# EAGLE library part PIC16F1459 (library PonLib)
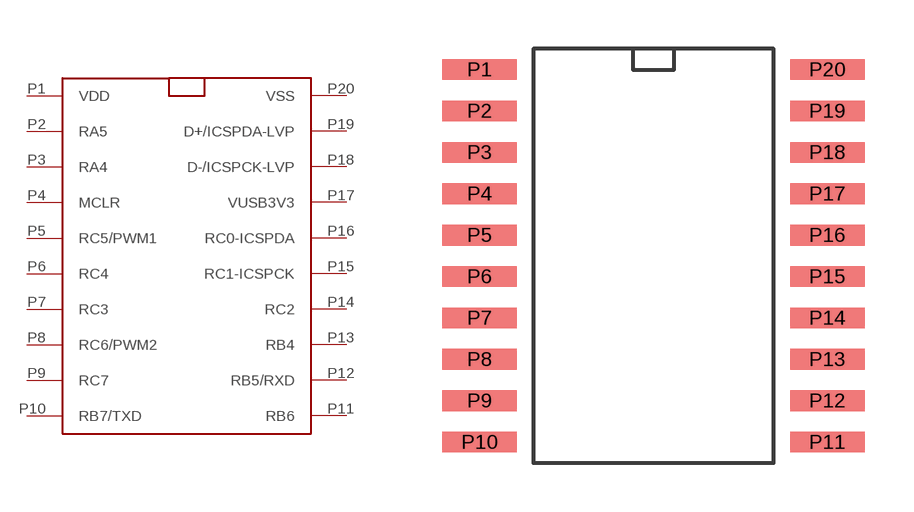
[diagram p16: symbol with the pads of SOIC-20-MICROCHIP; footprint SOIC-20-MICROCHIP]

Designator prefix -

## PIC16F1459  [SOIC-20-MICROCHIP]
P1  VDD
P2  RA5
P3  RA4
P4  MCLR
P5  RC5/PWM1
P6  RC4
P7  RC3
P8  RC6/PWM2
P9  RC7
P10  RB7/TXD
P11  RB6
P12  RB5/RXD
P13  RB4
P14  RC2
P15  RC1-ICSPCK
P16  RC0-ICSPDA
P17  VUSB3V3
P18  D-/ICSPCK-LVP
P19  D+/ICSPDA-LVP
P20  VSS

## Footprint SOIC-20-MICROCHIP (pad centres in mm)
smd 2.286 x 0.635: P1 -5.334,5.715; P2 -5.334,4.445; P3 -5.334,3.175; P4 -5.334,1.905; P5 -5.334,0.635; P6 -5.334,-0.635; P7 -5.334,-1.905; P8 -5.334,-3.175; P9 -5.334,-4.445; P10 -5.334,-5.715; P11 5.334,-5.715; P12 5.334,-4.445; P13 5.334,-3.175; P14 5.334,-1.905; P15 5.334,-0.635; P16 5.334,0.635; P17 5.334,1.905; P18 5.334,3.175; P19 5.334,4.445; P20 5.334,5.715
